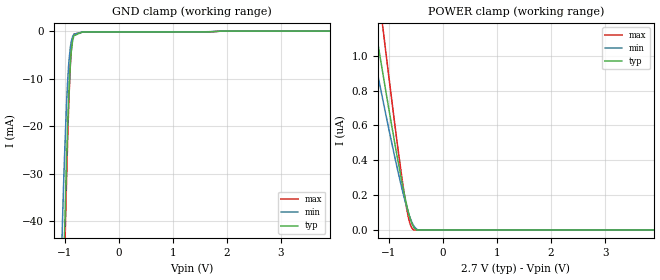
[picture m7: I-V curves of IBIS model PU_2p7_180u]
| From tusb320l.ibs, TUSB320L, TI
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|   Model
[Model]   PU_2p7_180u
Model_type   Input
Vinl = 0.81
Vinh = 1.89
|   typ   min   max
C_comp   0.475pF   0.451pF   0.489pF
[Voltage Range]   2.7   2.699   2.701
[Temperature Range]   27   105   -40
[Power Clamp Reference]   2.7   2.699   2.701
[GND Clamp Reference]   0   0   0
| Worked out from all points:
|   GND clamp passes 1 mA (typ) near -0.83 V on its own axis
[GND Clamp]
|   Voltage   I(typ)   I(min)   I(max)
-2.7V     -997.9mA   -935.8mA   -1.04A
-1.056V   -67.21mA   -46.46mA   -75.66mA
-1.04V    -59.5mA    -39.97mA   -67.28mA
-1.007V   -44.73mA   -28.03mA   -51.04mA
-966.6mV  -28mA      -15.7mA    -32.17mA
-942.3mV  -19.35mA   -10.1mA    -22.08mA
-918mV    -12.17mA   -6.029mA   -13.46mA
-893.7mV  -6.829mA   -3.372mA   -6.963mA
-877.5mV  -4.36mA    -2.238mA   -4.046mA
-828.9mV  -980.1uA   -671.6uA   -662.8uA
-666.9mV  -183.8uA   -166.6uA   -210.3uA
5.4V      0A         0A         0A
[POWER Clamp]
|   Voltage   I(typ)   I(min)   I(max)
-2.7V     3.977uA    3.304uA    5.388uA
-1.469V   1.576uA    1.306uA    2.096uA
-1.274V   1.206uA    999.7nA    1.586uA
-1.242V   1.145uA    949.1nA    1.502uA
-1.185V   1.038uA    861.2nA    1.354uA
-1.056V   797.1nA    663nA      1.022uA
-845.1mV  420nA      355.2nA    499.4nA
-666.9mV  138.9nA    128.9nA    117.6nA
-602.1mV  62.18nA    66.08nA    31.23nA
-537.3mV  15.04nA    22.98nA    0A
-464.4mV  0A         0A         0A
5.4V      0A         0A         0A
